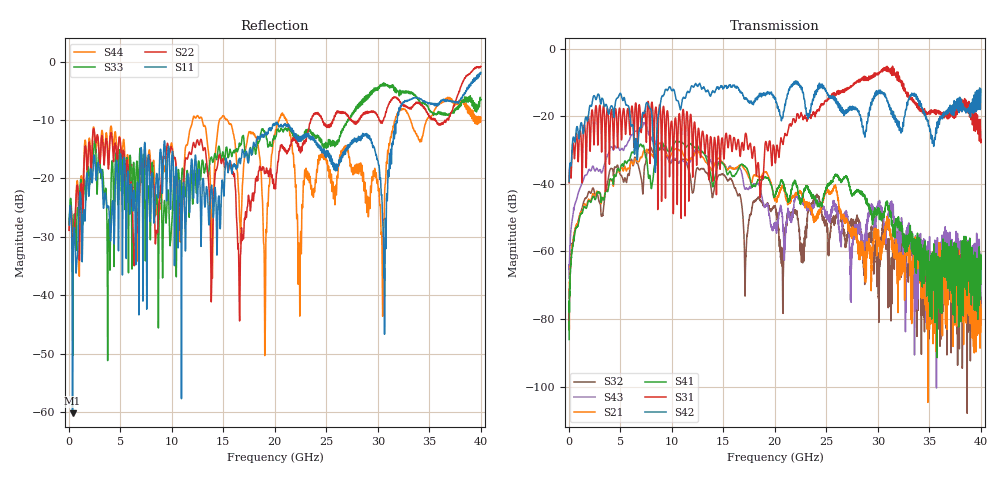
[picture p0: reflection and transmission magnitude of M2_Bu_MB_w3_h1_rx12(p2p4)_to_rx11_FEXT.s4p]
! S11 = S11
! S12 = S12
! S13 = S13
! S14 = S14
! S21 = S21
! S22 = S22
! S23 = S23
! S24 = S24
! S31 = S31
! S32 = S32
! S33 = S33
! S34 = S34
! S41 = S41
! S42 = S42
! S43 = S43
! S44 = S44
! FILE: \\englab.brocade.com\shares\Groups\SIT\Work\Shaohua\IEEE_channels\M2_Bu_MB_w3_h1_rx12(p2p4)_to_rx11_FEXT.s4p
!$DUT_CFG_DESC: Default 4-Port Configuration
!$NUMBER_PORTS: 4
!$DIFF_PORT_MAP: 1|2P|2|2P|0|UC|0|UC|
!$PORT_MAP: PNA 1|1|<<<<<<|TS 2|2|>>>>>>|PNA 2|3|<<<<<<|TS 4|4|>>>>>>|
# MHz S RI R 50.00
! FREQ  S11  S12  S13  S14
!  S21  S22  S23  S24
!  S31  S32  S33  S34
!  S41  S42  S43  S44
!  REAL  IMAG  REAL  IMAG  REAL  IMAG  REAL  IMAG
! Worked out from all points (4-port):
!   3996 points, 50 MHz to 40 GHz, reference 50 ohm
!   strongest paths, dB at 50 MHz, 10.04 GHz, 20.03 GHz, 30.02 GHz, 40 GHz:
!     S42: -39.3, -12.4, -14.8, -12.8, -12.0
!     S31: -39.6, -22.5, -33.3, -7.6, -26.9
!     S41: -86.1, -29.2, -43.3, -47.1, -60.9
!     S21: -83.3, -30.8, -44.9, -54.8, -75.8
!     S43: -67.9, -32.9, -53.2, -46.0, -68.0
!     S32: -71.1, -33.1, -47.0, -60.9, -73.5
!   lowest |S11| = -60.2 dB at 380 MHz (marker M1), VSWR 1.00, Z = 50.1 + j0.0573 ohm
!   |S11| at or under -10 dB: start of sweep to 31.88 GHz
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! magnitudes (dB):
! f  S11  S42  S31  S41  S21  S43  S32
! 50 MHz  -28.0  -39.3  -39.6  -86.1  -83.3  -67.9  -71.1
! 380 MHz  -60.2  -27.7  -28.5  -58.8  -57.8  -50.0  -58.0
! 8.93 GHz  -15.0  -15.8  -19.6  -29.2  -28.0  -29.3  -29.7
! 18.7 GHz  -12.8  -14.2  -39.5  -38.9  -37.8  -43.1  -45.4
! 30.63 GHz  -35.8  -13.1  -5.9  -48.2  -55.5  -53.1  -55.9
! 32.24 GHz  -7.7  -24.9  -9.3  -52.4  -62.5  -55.8  -66.3
! 40 GHz  -1.9  -12.0  -26.9  -60.9  -75.8  -68.0  -73.5
